| IBIS file stm32h523_533_ufbga100.ibs
[IBIS ver] 4.2
[File name] stm32h523_533_ufbga100.ibs
[File Rev] 0.2
[Date] 07-05-2024
[Source] Data Created at STMicroelectronics
[Notes]  File originated from ELDO simulations.
[Disclaimer]  This information is for modeling purpose only and is
   not guaranteed. The information is subject to change without
   notice.
[Copyright] Copyright 2024 STMicroelectronics Inc.
|   Component stm32h523_533_ufbga100
[Component] stm32h523_533_ufbga100
[Manufacturer] STMicroelectronics
[Package]
| variable   typ   min   max
R_pkg  0  NA  NA
L_pkg  0  NA  NA
C_pkg  0  NA  NA
[Pin]   signal_name   model_name
A1  PB9  io8_ft_i3c_spi
A2  PB8  io8_ft_i3c_spi
A3  BOOT0  vpphv
A4  PB5  io8_ft_i3c_spi
A5  PB3  io8_ft_i3c_spi
A6  PD6  io8_ft_i3c_spi
A7  PD4  io8_ft_i3c_spi
A8  PD3  io8_ft_i3c_spi
A9  PD1  io8_ft_i3c_spi
A10  PC11  io8_ft_i3c_spi
A11  PA15  io8_ft_i3c_spi
A12  PC10  io8_ft_i3c_spi
B1  PE0  io8_ft_i3c_spi
B2  PE4  io8_ft_i3c_spi
B3  PE3  io8_ft_i3c_spi
B4  PB6  io8_ft_i3c_spi
B5  PB4  io8_ft_i3c_spi
B6  PD7  io8_ft_i3c_spi
B7  PD5  io8_ft_i3c_spi
B8  PD2  io8_ft_i3c_spi
B9  PD0  io8_ft_i3c_spi
B10  PC12  io8_ft_i3c_spi
B11  PA14  io8_ft_i3c_spi
B12  PA13  io8_ft_i3c_spi
C1  PE2  io8_ft_i3c_spi
C2  PE5  io8_ft_i3c_spi
C3  VSS  gnd
C4  VCAP  nc
C5  PB7  io8_ft_i3c_spi
C8  VDDIO2  power
C9  VSS  gnd
C10  VDDUSB  power
C11  PA12  io8usb_ft_i3c_spi_phy
C12  PA11  io8usb_ft_i3c_spi_phy
D1  VBAT  power
D2  PE6  io8_ft_i3c_spi
D3  VDD  power
D10  VDD  power
D11  PA10  io8_ft_i3c_spi
D12  PA9  io8_ft_i3c_spi
E1  PC14-OSC32_IN  io_ft_tamp
E2  PC15-OSC32_OUT  io_ft_tamp
E3  PC13  io8_ft_i3c_spi_v33
E10  PA8  io8_ft_i3c_spi
E11  PC9  io8_ft_i3c_spi
E12  PC8  io8_ft_i3c_spi
F1  PH0-OSC_IN  io8_ft_i3c_spi
F2  PH1-OSC_OUT  io8_ft_i3c_spi
F11  PC7  io8_ft_i3c_spi
F12  PC6  io8_ft_i3c_spi
G1  PC0  io8_ft_spi
G2  NRST  ioreset_ft_v33
G11  PD14  io8_ft_i3c_spi
G12  PD15  io8_ft_i3c_spi
H1  PC2  io8_ft_spi
H2  PC3  io8_ft_spi
H3  PC1  io8_ft_spi
H10  PD11  io8_ft_i3c_spi
H11  PD12  io8_ft_i3c_spi
H12  PD13  io8_ft_i3c_spi
J1  VREFP  nc
J2  VSSA  nc
J3  VDD  power
J10  VDD  power
J11  PD9  io8_ft_i3c_spi
J12  PD10  io8_ft_i3c_spi
K1  VDDA  nc
K2  PA1  io8_ft_spi_tamp
K3  VSS  gnd
K4  PA2  io8_ft_spi
K5  PB1  io8_ft_spi
K8  PE12  io8_ft_i3c_spi
K9  VCAP  nc
K10  VSS  gnd
K11  PB14  nc
K12  PD8  io8_ft_i3c_spi
L1  PA3  io8_ft_spi
L2  PA4  io8_ft_spi
L3  PA0  io8_ft_spi
L4  PA7  io8_ft_spi
L5  PB2  io8_ft_i3c_spi
L6  VDD  power
L7  VSS  gnd
L8  PE10  io8_ft_i3c_spi
L9  PE13  io8_ft_i3c_spi
L10  PE15  io8_ft_i3c_spi
L11  PB12  io8_ft_i3c_spi
L12  PB15  io8_ft_spi
M1  PA6  io8_ft_spi
M2  PA5  io8_ft_spi
M3  PC4  io8_ft_spi
M4  PC5  io8_ft_spi
M5  PB0  io8_ft_spi
M6  PE7  io8_ft_i3c_spi
M7  PE8  io8_ft_i3c_spi
M8  PE9  io8_ft_i3c_spi
M9  PE11  io8_ft_i3c_spi
M10  PE14  io8_ft_i3c_spi
M11  PB10  io8_ft_i3c_spi
M12  PB13  nc
[Package Model]   478-ufbga7x7-100-240126
[Pin Mapping]   pulldown_ref   pullup_ref   | Comment
A1  gndio  vddmmc
A2  gndio  vddmmc
A3  gndio  vddio
A4  gndio  vddio
A5  gndio  vddio
A6  gndio  vddmmc
A7  gndio  vddio
A8  gndio  vddio
A9  gndio  vddio
A10  gndio  vddio
A11  gndio  vddio
A12  gndio  vddio
B1  gndio  vddio
B2  gndio  vddio
B3  gndio  vddio
B4  gndio  vddio
B5  gndio  vddio
B6  gndio  vddmmc
B7  gndio  vddio
B8  gndio  vddio
B9  gndio  vddio
B10  gndio  vddio
B11  gndio  vddio
B12  gndio  vddio
C1  gndio  vddio
C2  gndio  vddio
C3  gndio  nc
C4  nc  nc
C5  gndio  vddio
C8  nc  vddmmc
C9  gndio  nc
C10  nc  vddusb
C11  gndio  vddusb  | Depending on IO usage
| C11  gndio  vddio  | Depending on IO usage
C12  gndio  vddusb  | Depending on IO usage
| C12  gndio  vddio  | Depending on IO usage
D1  nc  vsw
D2  gndio  vddio
D3  nc  vddio
D10  nc  vddio
D11  gndio  vddio
D12  gndio  vddio
E1  gndio  vddio  | Depending on IO usage
| E1  gndio  vsw  | Depending on IO usage
E2  gndio  vddio  | Depending on IO usage
| E2  gndio  vsw  | Depending on IO usage
E3  gndio  vddio  | Depending on IO usage
| E3  gndio  vsw  | Depending on IO usage
E10  gndio  vddio
E11  gndio  vddio
E12  gndio  vddio
F1  gndio  vddio
F2  gndio  vddio
F11  gndio  vddio
F12  gndio  vddio
G1  gndio  vddio
G2  gndio  vddio
G11  gndio  vddio
G12  gndio  vddio
H1  gndio  vddio
H2  gndio  vddio
H3  gndio  vddio
H10  gndio  vddio
H11  gndio  vddio
H12  gndio  vddio
J1  nc  nc
J2  nc  nc
J3  nc  vddio
J10  nc  vddio
J11  gndio  vddio
J12  gndio  vddio
K1  nc  nc
K2  gndio  vddio
K3  gndio  nc
K4  gndio  vddio
K5  gndio  vddio
K8  gndio  vddio
K9  nc  nc
K10  gndio  nc
K11  nc  nc
K12  gndio  vddio
L1  gndio  vddio
L2  gndio  vddio
L3  gndio  vddio
L4  gndio  vddio
L5  gndio  vddio
L6  nc  vddio
L7  gndio  nc
L8  gndio  vddio
L9  gndio  vddio
L10  gndio  vddio
L11  gndio  vddio
L12  gndio  vddio
M1  gndio  vddio
M2  gndio  vddio
M3  gndio  vddio
M4  gndio  vddio
M5  gndio  vddio
M6  gndio  vddio
M7  gndio  vddio
M8  gndio  vddio
M9  gndio  vddio
M10  gndio  vddio
M11  gndio  vddio
M12  nc  nc
|[Diff Pin]  inv_pin  vdiff  tdelay_typ  tdelay_min  tdelay_max
|C11  C12  NA  NA  NA  NA
[Model Selector] io8_ft_i3c_spi
io8_ft_spi_ls_1v2 "GPIO SPI - 5V tolerant - low speed - 1.2V range"
io8_ft_spi_ls_1v8 "GPIO SPI - 5V tolerant - low speed - 1.8V range"
io8_ft_spi_ls_3v3 "GPIO SPI - 5V tolerant - low speed - 3.3V range"
io8_ft_spi_ms_1v2 "GPIO SPI - 5V tolerant - med speed - 1.2V range"
io8_ft_spi_ms_1v8 "GPIO SPI - 5V tolerant - med speed - 1.8V range"
io8_ft_spi_ms_3v3 "GPIO SPI - 5V tolerant - med speed - 3.3V range"
io8_ft_spi_fs_1v2 "GPIO SPI - 5V tolerant - fast speed - 1.2V range"
io8_ft_spi_fs_1v8 "GPIO SPI - 5V tolerant - fast speed - 1.8V range"
io8_ft_spi_fs_3v3 "GPIO SPI - 5V tolerant - fast speed - 3.3V range"
io8_ft_spi_hs_1v2 "GPIO SPI - 5V tolerant - high speed - 1.2V range"
io8_ft_spi_hs_1v8 "GPIO SPI - 5V tolerant - high speed - 1.8V range"
io8_ft_spi_hs_3v3 "GPIO SPI - 5V tolerant - high speed - 3.3V range"
io8_ft_hslv_spi_ls_1v2 "GPIO SPI low volt opt - 5V tolerant - low speed - 1.2V range"
io8_ft_hslv_spi_ls_1v8 "GPIO SPI low volt opt - 5V tolerant - low speed - 1.8V range"
io8_ft_hslv_spi_ls_2v5 "GPIO SPI low volt opt - 5V tolerant - low speed - 2.5V range"
io8_ft_hslv_spi_ms_1v2 "GPIO SPI low volt opt - 5V tolerant - med speed - 1.2V range"
io8_ft_hslv_spi_ms_1v8 "GPIO SPI low volt opt - 5V tolerant - med speed - 1.8V range"
io8_ft_hslv_spi_ms_2v5 "GPIO SPI low volt opt - 5V tolerant - med speed - 2.5V range"
io8_ft_hslv_spi_fs_1v2 "GPIO SPI low volt opt - 5V tolerant - fast speed - 1.2V range"
io8_ft_hslv_spi_fs_1v8 "GPIO SPI low volt opt - 5V tolerant - fast speed - 1.8V range"
io8_ft_hslv_spi_fs_2v5 "GPIO SPI low volt opt - 5V tolerant - fast speed - 2.5V range"
io8_ft_hslv_spi_hs_1v2 "GPIO SPI low volt opt - 5V tolerant - high speed - 1.2V range"
io8_ft_hslv_spi_hs_1v8 "GPIO SPI low volt opt - 5V tolerant - high speed - 1.8V range"
io8_ft_hslv_spi_hs_2v5 "GPIO SPI low volt opt - 5V tolerant - high speed - 2.5V range"
io8_ft_i3c_spi_ls_1v2 "GPIO SPI with I3C open-drain - 5V tolerant - low speed - 1.2V range"
io8_ft_i3c_spi_ls_1v8 "GPIO SPI with I3C open-drain - 5V tolerant - low speed - 1.8V range"
io8_ft_i3c_spi_ls_3v3 "GPIO SPI with I3C open-drain - 5V tolerant - low speed - 3.3V range"
io8_ft_i3c_spi_ms_1v2 "GPIO SPI with I3C open-drain - 5V tolerant - med speed - 1.2V range"
io8_ft_i3c_spi_ms_1v8 "GPIO SPI with I3C open-drain - 5V tolerant - med speed - 1.8V range"
io8_ft_i3c_spi_ms_3v3 "GPIO SPI with I3C open-drain - 5V tolerant - med speed - 3.3V range"
io8_ft_i3c_spi_fs_1v2 "GPIO SPI with I3C open-drain - 5V tolerant - fast speed - 1.2V range"
io8_ft_i3c_spi_fs_1v8 "GPIO SPI with I3C open-drain - 5V tolerant - fast speed - 1.8V range"
io8_ft_i3c_spi_fs_3v3 "GPIO SPI with I3C open-drain - 5V tolerant - fast speed - 3.3V range"
io8_ft_i3c_spi_hs_1v2 "GPIO SPI with I3C open-drain - 5V tolerant - high speed - 1.2V range"
io8_ft_i3c_spi_hs_1v8 "GPIO SPI with I3C open-drain - 5V tolerant - high speed - 1.8V range"
io8_ft_i3c_spi_hs_3v3 "GPIO SPI with I3C open-drain - 5V tolerant - high speed - 3.3V range"
io8_ft_hslv_i3c_spi_ls_1v2 "GPIO SPI low volt opt with I3C open-drain - 5V tolerant - low speed - 1.2V range"
io8_ft_hslv_i3c_spi_ls_1v8 "GPIO SPI low volt opt with I3C open-drain - 5V tolerant - low speed - 1.8V range"
io8_ft_hslv_i3c_spi_ls_2v5 "GPIO SPI low volt opt with I3C open-drain - 5V tolerant - low speed - 2.5V range"
io8_ft_hslv_i3c_spi_ms_1v2 "GPIO SPI low volt opt with I3C open-drain - 5V tolerant - med speed - 1.2V range"
io8_ft_hslv_i3c_spi_ms_1v8 "GPIO SPI low volt opt with I3C open-drain - 5V tolerant - med speed - 1.8V range"
io8_ft_hslv_i3c_spi_ms_2v5 "GPIO SPI low volt opt with I3C open-drain - 5V tolerant - med speed - 2.5V range"
io8_ft_hslv_i3c_spi_fs_1v2 "GPIO SPI low volt opt with I3C open-drain - 5V tolerant - fast speed - 1.2V range"
io8_ft_hslv_i3c_spi_fs_1v8 "GPIO SPI low volt opt with I3C open-drain - 5V tolerant - fast speed - 1.8V range"
io8_ft_hslv_i3c_spi_fs_2v5 "GPIO SPI low volt opt with I3C open-drain - 5V tolerant - fast speed - 2.5V range"
io8_ft_hslv_i3c_spi_hs_1v2 "GPIO SPI low volt opt with I3C open-drain - 5V tolerant - high speed - 1.2V range"
io8_ft_hslv_i3c_spi_hs_1v8 "GPIO SPI low volt opt with I3C open-drain - 5V tolerant - high speed - 1.8V range"
io8_ft_hslv_i3c_spi_hs_2v5 "GPIO SPI low volt opt with I3C open-drain - 5V tolerant - high speed - 2.5V range"
io8_ft_i3c_fmp_spi_3v3 "GPIO SPI with I3C fm+ open-drain - 5V tolerant - 3.3V range"
io8_ft_i3c_fmp_spi_1v8 "GPIO SPI with I3C fm+ open-drain - 5V tolerant - 1.8V range"
io8_ft_i3c_fmp_spi_1v2 "GPIO SPI with I3C fm+ open-drain - 5V tolerant - 1.2V range"
[Model Selector] io8_ft_i3c_spi_v33
io8_ft_spi_v33_ls_1v2 ""GPIO SPI V33 - 5V tolerant - low speed - 1.2V range"
io8_ft_spi_v33_ls_1v8 ""GPIO SPI V33 - 5V tolerant - low speed - 1.8V range"
io8_ft_spi_v33_ls_3v3 ""GPIO SPI V33 - 5V tolerant - low speed - 3.3V range"
io8_ft_spi_v33_ms_1v2 ""GPIO SPI V33 - 5V tolerant - med speed - 1.2V range"
io8_ft_spi_v33_ms_1v8 ""GPIO SPI V33 - 5V tolerant - med speed - 1.8V range"
io8_ft_spi_v33_ms_3v3 ""GPIO SPI V33 - 5V tolerant - med speed - 3.3V range"
io8_ft_spi_v33_fs_1v2 ""GPIO SPI V33 - 5V tolerant - fast speed - 1.2V range
io8_ft_spi_v33_fs_1v8 ""GPIO SPI V33 - 5V tolerant - fast speed - 1.8V range
io8_ft_spi_v33_fs_3v3 ""GPIO SPI V33 - 5V tolerant - fast speed - 3.3V range
io8_ft_spi_v33_hs_1v2 ""GPIO SPI V33 - 5V tolerant - high speed - 1.2V range
io8_ft_spi_v33_hs_1v8 ""GPIO SPI V33 - 5V tolerant - high speed - 1.8V range
io8_ft_spi_v33_hs_3v3 ""GPIO SPI V33 - 5V tolerant - high speed - 3.3V range
io8_ft_hslv_spi_v33_ls_1v2 "GPIO SPI V33 low volt opt - 5V tolerant - low speed - 1.2V range""
io8_ft_hslv_spi_v33_ls_1v8 "GPIO SPI V33 low volt opt - 5V tolerant - low speed - 1.8V range""
io8_ft_hslv_spi_v33_ls_2v5 "GPIO SPI V33 low volt opt - 5V tolerant - low speed - 2.5V range""
io8_ft_hslv_spi_v33_ms_1v2 "GPIO SPI V33 low volt opt - 5V tolerant - med speed - 1.2V range""
io8_ft_hslv_spi_v33_ms_1v8 "GPIO SPI V33 low volt opt - 5V tolerant - med speed - 1.8V range""
io8_ft_hslv_spi_v33_ms_2v5 "GPIO SPI V33 low volt opt - 5V tolerant - med speed - 2.5V range""
io8_ft_hslv_spi_v33_fs_1v2 "GPIO SPI V33 low volt opt - 5V tolerant - fast speed - 1.2V range"
io8_ft_hslv_spi_v33_fs_1v8 "GPIO SPI V33 low volt opt - 5V tolerant - fast speed - 1.8V range"
io8_ft_hslv_spi_v33_fs_2v5 "GPIO SPI V33 low volt opt - 5V tolerant - fast speed - 2.5V range"
io8_ft_hslv_spi_v33_hs_1v2 "GPIO SPI V33 low volt opt - 5V tolerant - high speed - 1.2V range"
io8_ft_hslv_spi_v33_hs_1v8 "GPIO SPI V33 low volt opt - 5V tolerant - high speed - 1.8V range"
io8_ft_hslv_spi_v33_hs_2v5 "GPIO SPI V33 low volt opt - 5V tolerant - high speed - 2.5V range"
io8_ft_i3c_spi_v33_ls_1v2 "GPIO SPI V33 with I3C open-drain - 5V tolerant - low speed - 1.2V range"
io8_ft_i3c_spi_v33_ls_1v8 "GPIO SPI V33 with I3C open-drain - 5V tolerant - low speed - 1.8V range"
io8_ft_i3c_spi_v33_ls_3v3 "GPIO SPI V33 with I3C open-drain - 5V tolerant - low speed - 3.3V range"
io8_ft_i3c_spi_v33_ms_1v2 "GPIO SPI V33 with I3C open-drain - 5V tolerant - med speed - 1.2V range"
io8_ft_i3c_spi_v33_ms_1v8 "GPIO SPI V33 with I3C open-drain - 5V tolerant - med speed - 1.8V range"
io8_ft_i3c_spi_v33_ms_3v3 "GPIO SPI V33 with I3C open-drain - 5V tolerant - med speed - 3.3V range"
io8_ft_i3c_spi_v33_fs_1v2 "GPIO SPI V33 with I3C open-drain - 5V tolerant - fast speed - 1.2V range"
io8_ft_i3c_spi_v33_fs_1v8 "GPIO SPI V33 with I3C open-drain - 5V tolerant - fast speed - 1.8V range"
io8_ft_i3c_spi_v33_fs_3v3 "GPIO SPI V33 with I3C open-drain - 5V tolerant - fast speed - 3.3V range"
io8_ft_i3c_spi_v33_hs_1v2 "GPIO SPI V33 with I3C open-drain - 5V tolerant - high speed - 1.2V range"
io8_ft_i3c_spi_v33_hs_1v8 "GPIO SPI V33 with I3C open-drain - 5V tolerant - high speed - 1.8V range"
io8_ft_i3c_spi_v33_hs_3v3 "GPIO SPI V33 with I3C open-drain - 5V tolerant - high speed - 3.3V range"
io8_ft_hslv_i3c_spi_v33_ls_1v2 "GPIO SPI V33 low volt opt with I3C open-drain - 5V tolerant - low speed - 1.2V range"
io8_ft_hslv_i3c_spi_v33_ls_1v8 "GPIO SPI V33 low volt opt with I3C open-drain - 5V tolerant - low speed - 1.8V range"
io8_ft_hslv_i3c_spi_v33_ls_2v5 "GPIO SPI V33 low volt opt with I3C open-drain - 5V tolerant - low speed - 2.5V range"
io8_ft_hslv_i3c_spi_v33_ms_1v2 "GPIO SPI V33 low volt opt with I3C open-drain - 5V tolerant - med speed - 1.2V range"
io8_ft_hslv_i3c_spi_v33_ms_1v8 "GPIO SPI V33 low volt opt with I3C open-drain - 5V tolerant - med speed - 1.8V range"
io8_ft_hslv_i3c_spi_v33_ms_2v5 "GPIO SPI V33 low volt opt with I3C open-drain - 5V tolerant - med speed - 2.5V range"
io8_ft_hslv_i3c_spi_v33_fs_1v2 "GPIO SPI V33 low volt opt with I3C open-drain - 5V tolerant - fast speed - 1.2V range"
io8_ft_hslv_i3c_spi_v33_fs_1v8 "GPIO SPI V33 low volt opt with I3C open-drain - 5V tolerant - fast speed - 1.8V range"
io8_ft_hslv_i3c_spi_v33_fs_2v5 "GPIO SPI V33 low volt opt with I3C open-drain - 5V tolerant - fast speed - 2.5V range"
io8_ft_hslv_i3c_spi_v33_hs_1v2 "GPIO SPI V33 low volt opt with I3C open-drain - 5V tolerant - high speed - 1.2V range"
io8_ft_hslv_i3c_spi_v33_hs_1v8 "GPIO SPI V33 low volt opt with I3C open-drain - 5V tolerant - high speed - 1.8V range"
io8_ft_hslv_i3c_spi_v33_hs_2v5 "GPIO SPI V33 low volt opt with I3C open-drain - 5V tolerant - high speed - 2.5V range"
io8_ft_i3c_fmp_spi_v33_3v3 "GPIO SPI V33 with I3C fm+ open-drain - 5V tolerant - 3.3V range"
io8_ft_i3c_fmp_spi_v33_1v8 "GPIO SPI V33 with I3C fm+ open-drain - 5V tolerant - 1.8V range"
io8_ft_i3c_fmp_spi_v33_1v2 "GPIO SPI V33 with I3C fm+ open-drain - 5V tolerant - 1.2V range"
[Model Selector] io8_ft_spi
io8_ft_spi_ls_1v2 "GPIO SPI - 5V tolerant - low speed - 1.2V range"
io8_ft_spi_ls_1v8 "GPIO SPI - 5V tolerant - low speed - 1.8V range"
io8_ft_spi_ls_3v3 "GPIO SPI - 5V tolerant - low speed - 3.3V range"
io8_ft_spi_ms_1v2 "GPIO SPI- 5V tolerant - med speed - 1.2V range"
io8_ft_spi_ms_1v8 "GPIO SPI- 5V tolerant - med speed - 1.8V range"
io8_ft_spi_ms_3v3 "GPIO SPI- 5V tolerant - med speed - 3.3V range"
io8_ft_spi_fs_1v2 "GPIO SPI- 5V tolerant - fast speed - 1.2V range"
io8_ft_spi_fs_1v8 "GPIO SPI- 5V tolerant - fast speed - 1.8V range"
io8_ft_spi_fs_3v3 "GPIO SPI- 5V tolerant - fast speed - 3.3V range"
io8_ft_spi_hs_1v2 "GPIO SPI- 5V tolerant - high speed - 1.2V range"
io8_ft_spi_hs_1v8 "GPIO SPI- 5V tolerant - high speed - 1.8V range"
io8_ft_spi_hs_3v3 "GPIO SPI- 5V tolerant - high speed - 3.3V range"
io8_ft_hslv_spi_ls_1v2 "GPIO SPI low volt opt - 5V tolerant - low speed - 1.2V range"
io8_ft_hslv_spi_ls_1v8 "GPIO SPI low volt opt - 5V tolerant - low speed - 1.8V range"
io8_ft_hslv_spi_ls_2v5 "GPIO SPI low volt opt - 5V tolerant - low speed - 2.5V range"
io8_ft_hslv_spi_ms_1v2 "GPIO SPI low volt opt - 5V tolerant - med speed - 1.2V range"
io8_ft_hslv_spi_ms_1v8 "GPIO SPI low volt opt - 5V tolerant - med speed - 1.8V range"
io8_ft_hslv_spi_ms_2v5 "GPIO SPI low volt opt - 5V tolerant - med speed - 2.5V range"
io8_ft_hslv_spi_fs_1v2 "GPIO SPI low volt opt - 5V tolerant - fast speed - 1.2V range"
io8_ft_hslv_spi_fs_1v8 "GPIO SPI low volt opt - 5V tolerant - fast speed - 1.8V range"
io8_ft_hslv_spi_fs_2v5 "GPIO SPI low volt opt - 5V tolerant - fast speed - 2.5V range"
io8_ft_hslv_spi_hs_1v2 "GPIO SPI low volt opt - 5V tolerant - high speed - 1.2V range"
io8_ft_hslv_spi_hs_1v8 "GPIO SPI low volt opt - 5V tolerant - high speed - 1.8V range"
io8_ft_hslv_spi_hs_2v5 "GPIO SPI low volt opt - 5V tolerant - high speed - 2.5V range"
[Model Selector] io8_ft_spi_tamp
io8_ft_spi_ls_1v2 "GPIO SPI - 5V tolerant - low speed - 1.2V range"
io8_ft_spi_ls_1v8 "GPIO SPI - 5V tolerant - low speed - 1.8V range"
io8_ft_spi_ls_3v3 "GPIO SPI- 5V tolerant - low speed - 3.3V range"
io8_ft_spi_ms_1v2 "GPIO SPI - 5V tolerant - med speed - 1.2V range"
io8_ft_spi_ms_1v8 "GPIO SPI - 5V tolerant - med speed - 1.8V range"
io8_ft_spi_ms_3v3 "GPIO SPI - 5V tolerant - med speed - 3.3V range"
io8_ft_spi_fs_1v2 "GPIO SPI - 5V tolerant - fast speed - 1.2V range"
io8_ft_spi_fs_1v8 "GPIO SPI - 5V tolerant - fast speed - 1.8V range"
io8_ft_spi_fs_3v3 "GPIO SPI - 5V tolerant - fast speed - 3.3V range"
io8_ft_spi_hs_1v2 "GPIO SPI - 5V tolerant - high speed - 1.2V range"
io8_ft_spi_hs_1v8 "GPIO SPI - 5V tolerant - high speed - 1.8V range"
io8_ft_spi_hs_3v3 "GPIO SPI - 5V tolerant - high speed - 3.3V range"
io8_ft_hslv_spi_ls_1v2 "GPIO SPI low volt opt - 5V tolerant - low speed - 1.2V range"
io8_ft_hslv_spi_ls_1v8 "GPIO SPI low volt opt - 5V tolerant - low speed - 1.8V range"
io8_ft_hslv_spi_ls_2v5 "GPIO SPI low volt opt - 5V tolerant - low speed - 2.5V range"
io8_ft_hslv_spi_ms_1v2 "GPIO SPI low volt opt - 5V tolerant - med speed - 1.2V range"
io8_ft_hslv_spi_ms_1v8 "GPIO SPI low volt opt - 5V tolerant - med speed - 1.8V range"
io8_ft_hslv_spi_ms_2v5 "GPIO SPI low volt opt - 5V tolerant - med speed - 2.5V range"
io8_ft_hslv_spi_fs_1v2 "GPIO SPI low volt opt - 5V tolerant - fast speed - 1.2V range"
io8_ft_hslv_spi_fs_1v8 "GPIO SPI low volt opt - 5V tolerant - fast speed - 1.8V range"
io8_ft_hslv_spi_fs_2v5 "GPIO SPI low volt opt - 5V tolerant - fast speed - 2.5V range"
io8_ft_hslv_spi_hs_1v2 "GPIO SPI low volt opt - 5V tolerant - high speed - 1.2V range"
io8_ft_hslv_spi_hs_1v8 "GPIO SPI low volt opt - 5V tolerant - high speed - 1.8V range"
io8_ft_hslv_spi_hs_2v5 "GPIO SPI low volt opt - 5V tolerant - high speed - 2.5V range
io8_ft_tamp_v33_1v2 "IO tamper - 5V tolerant - 1.2V range"
io8_ft_tamp_v33_1v8 "IO tamper - 5V tolerant - 1.8V range"
io8_ft_tamp_v33_3v3 "IO tamper - 5V tolerant - 3.3V range"
[Model Selector] io8usb_ft_i3c_spi_phy
io8_ft_spi_ls_1v2 "GPIO SPI - 5V tolerant - low speed - 1.2V range"
io8_ft_spi_ls_1v8 "GPIO SPI - 5V tolerant - low speed - 1.8V range"
io8_ft_spi_ls_3v3 "GPIO SPI - 5V tolerant - low speed - 3.3V range"
io8_ft_spi_ms_1v2 "GPIO SPI - 5V tolerant - med speed - 1.2V range"
io8_ft_spi_ms_1v8 "GPIO SPI - 5V tolerant - med speed - 1.8V range"
io8_ft_spi_ms_3v3 "GPIO SPI - 5V tolerant - med speed - 3.3V range"
io8_ft_spi_fs_1v2 "GPIO SPI - 5V tolerant - fast speed - 1.2V range"
io8_ft_spi_fs_1v8 "GPIO SPI - 5V tolerant - fast speed - 1.8V range"
io8_ft_spi_fs_3v3 "GPIO SPI - 5V tolerant - fast speed - 3.3V range"
io8_ft_spi_hs_1v2 "GPIO SPI - 5V tolerant - high speed - 1.2V range"
io8_ft_spi_hs_1v8 "GPIO SPI - 5V tolerant - high speed - 1.8V range"
io8_ft_spi_hs_3v3 "GPIO SPI - 5V tolerant - high speed - 3.3V range"
io8_ft_hslv_spi_ls_1v2 "GPIO SPI low volt opt - 5V tolerant - low speed - 1.2V range"
io8_ft_hslv_spi_ls_1v8 "GPIO SPI low volt opt - 5V tolerant - low speed - 1.8V range"
io8_ft_hslv_spi_ls_2v5 "GPIO SPI low volt opt - 5V tolerant - low speed - 2.5V range"
io8_ft_hslv_spi_ms_1v2 "GPIO SPI low volt opt - 5V tolerant - med speed - 1.2V range"
io8_ft_hslv_spi_ms_1v8 "GPIO SPI low volt opt - 5V tolerant - med speed - 1.8V range"
io8_ft_hslv_spi_ms_2v5 "GPIO SPI low volt opt - 5V tolerant - med speed - 2.5V range"
io8_ft_hslv_spi_fs_1v2 "GPIO SPI low volt opt - 5V tolerant - fast speed - 1.2V range"
io8_ft_hslv_spi_fs_1v8 "GPIO SPI low volt opt - 5V tolerant - fast speed - 1.8V range"
io8_ft_hslv_spi_fs_2v5 "GPIO SPI low volt opt - 5V tolerant - fast speed - 2.5V range"
io8_ft_hslv_spi_hs_1v2 "GPIO SPI low volt opt - 5V tolerant - high speed - 1.2V range"
io8_ft_hslv_spi_hs_1v8 "GPIO SPI low volt opt - 5V tolerant - high speed - 1.8V range"
io8_ft_hslv_spi_hs_2v5 "GPIO SPI low volt opt - 5V tolerant - high speed - 2.5V range"
io8_ft_i3c_spi_ls_1v2 "GPIO SPI  with I3C open-drain - 5V tolerant - low speed - 1.2V range"
io8_ft_i3c_spi_ls_1v8 "GPIO SPI  with I3C open-drain - 5V tolerant - low speed - 1.8V range"
io8_ft_i3c_spi_ls_3v3 "GPIO SPI  with I3C open-drain - 5V tolerant - low speed - 3.3V range"
io8_ft_i3c_spi_ms_1v2 "GPIO SPI  with I3C open-drain - 5V tolerant - med speed - 1.2V range"
io8_ft_i3c_spi_ms_1v8 "GPIO SPI  with I3C open-drain - 5V tolerant - med speed - 1.8V range"
io8_ft_i3c_spi_ms_3v3 "GPIO SPI  with I3C open-drain - 5V tolerant - med speed - 3.3V range"
io8_ft_i3c_spi_fs_1v2 "GPIO SPI  with I3C open-drain - 5V tolerant - fast speed - 1.2V range"
io8_ft_i3c_spi_fs_1v8 "GPIO SPI  with I3C open-drain - 5V tolerant - fast speed - 1.8V range"
io8_ft_i3c_spi_fs_3v3 "GPIO SPI  with I3C open-drain - 5V tolerant - fast speed - 3.3V range"
io8_ft_i3c_spi_hs_1v2 "GPIO SPI  with I3C open-drain - 5V tolerant - high speed - 1.2V range"
io8_ft_i3c_spi_hs_1v8 "GPIO SPI  with I3C open-drain - 5V tolerant - high speed - 1.8V range"
io8_ft_i3c_spi_hs_3v3 "GPIO SPI  with I3C open-drain - 5V tolerant - high speed - 3.3V range"
io8_ft_hslv_i3c_spi_ls_1v2 "GPIO SPI  low volt opt with I3C open-drain - 5V tolerant - low speed - 1.2V range"
io8_ft_hslv_i3c_spi_ls_1v8 "GPIO SPI  low volt opt with I3C open-drain - 5V tolerant - low speed - 1.8V range"
io8_ft_hslv_i3c_spi_ls_2v5 "GPIO SPI  low volt opt with I3C open-drain - 5V tolerant - low speed - 2.5V range"
io8_ft_hslv_i3c_spi_ms_1v2 "GPIO SPI  low volt opt with I3C open-drain - 5V tolerant - med speed - 1.2V range"
io8_ft_hslv_i3c_spi_ms_1v8 "GPIO SPI  low volt opt with I3C open-drain - 5V tolerant - med speed - 1.8V range"
io8_ft_hslv_i3c_spi_ms_2v5 "GPIO SPI  low volt opt with I3C open-drain - 5V tolerant - med speed - 2.5V range"
io8_ft_hslv_i3c_spi_fs_1v2 "GPIO SPI  low volt opt with I3C open-drain - 5V tolerant - fast speed - 1.2V range"
io8_ft_hslv_i3c_spi_fs_1v8 "GPIO SPI  low volt opt with I3C open-drain - 5V tolerant - fast speed - 1.8V range"
io8_ft_hslv_i3c_spi_fs_2v5 "GPIO SPI  low volt opt with I3C open-drain - 5V tolerant - fast speed - 2.5V range"
io8_ft_hslv_i3c_spi_hs_1v2 "GPIO SPI  low volt opt with I3C open-drain - 5V tolerant - high speed - 1.2V range"
io8_ft_hslv_i3c_spi_hs_1v8 "GPIO SPI  low volt opt with I3C open-drain - 5V tolerant - high speed - 1.8V range"
io8_ft_hslv_i3c_spi_hs_2v5 "GPIO SPI  low volt opt with I3C open-drain - 5V tolerant - high speed - 2.5V range"
io8_ft_i3c_fmp_spi_3v3 "GPIO SPI  with I3C fm+ open-drain - 5V tolerant - 3.3V range"
io8_ft_i3c_fmp_spi_1v8 "GPIO SPI  with I3C fm+ open-drain - 5V tolerant - 1.8V range"
io8_ft_i3c_fmp_spi_1v2 "GPIO SPI  with I3C fm+ open-drain - 5V tolerant - 1.2V range"
io8usb_ft_phy_ls_2v5 "USB PHY - 5V tolerant - low speed - 2.5V range"
io8usb_ft_phy_ls_3v3 "USB PHY - 5V tolerant - low speed - 3.3V range
io8usb_ft_phy_fs_2v5 "USB PHY - 5V tolerant - fast speed - 2.5V range"
io8usb_ft_phy_fs_3v3 "USB PHY - 5V tolerant - fast speed - 3.3V range"
[Model Selector] io_ft_tamp
io_ft_tamp_3v3 "IO tamper - 5V tolerant - 3.3V range"
io_ft_tamp_1v8 "IO tamper - 5V tolerant - 1.8V range"
io_ft_tamp_1v2 "IO tamper - 5V tolerant - 1.2V range"
[Model Selector] ioreset_ft_v33
ioreset_ft_v33_1v2 "Reset PAD. 5V tolerant. 1.2V range"
ioreset_ft_v33_1v8 "Reset PAD. 5V tolerant. 1.8V range"
ioreset_ft_v33_3v3 "Reset PAD. 5V tolerant. 3.3V range"
[Model Selector] vpphv
vpphv_1v2 "Flash Test cell v33 = 1.2 V range"
vpphv_1v8 "Flash Test cell v33 = 1.8 V range"
vpphv_3v3 "Flash Test cell v33 = 3.3 V range"
[Define Package Model]  478-ufbga7x7-100-240126
[Manufacturer]  unknown
[OEM]  unknown
[Description]  unknown
[Number Of Pins]  92
[Pin Numbers]
| Pin Name Terminal   Net Name   Starting Node   Ending Node
A3 | BOOT0
G2 | NRST
L3 | PA0
K2 | PA1
K4 | PA2
L1 | PA3
L2 | PA4
M2 | PA5
M1 | PA6
L4 | PA7
E10 | PA8
D12 | PA9
D11 | PA10
C12 | PA11
C11 | PA12
B12 | PA13
B11 | PA14
A11 | PA15
M5 | PB0
K5 | PB1
L5 | PB2
A5 | PB3
B5 | PB4
A4 | PB5
B4 | PB6
C5 | PB7
A2 | PB8
A1 | PB9
M11 | PB10
L11 | PB12
M12 | PB13
K11 | PB14
L12 | PB15
G1 | PC0
H3 | PC1
H1 | PC2
H2 | PC3
M3 | PC4
M4 | PC5
F12 | PC6
F11 | PC7
E12 | PC8
E11 | PC9
A12 | PC10
A10 | PC11
B10 | PC12
E3 | PC13
E1 | PC14-OSC32_IN
E2 | PC15-OSC32_OUT
B9 | PD0
A9 | PD1
B8 | PD2
A8 | PD3
A7 | PD4
B7 | PD5
A6 | PD6
B6 | PD7
K12 | PD8
J11 | PD9
J12 | PD10
H10 | PD11
H11 | PD12
H12 | PD13
G11 | PD14
G12 | PD15
B1 | PE0
C1 | PE2
B3 | PE3
B2 | PE4
C2 | PE5
D2 | PE6
M6 | PE7
M7 | PE8
M8 | PE9
L8 | PE10
M9 | PE11
K8 | PE12
L9 | PE13
M10 | PE14
L10 | PE15
F1 | PH0-OSC_IN
F2 | PH1-OSC_OUT
D1 | VBAT
K9 | VCAP
C4 | VCAP
D3 | VDD
K1 | VDDA
C8 | VDDIO2
C10 | VDDUSB
J1 | VREFP
C3 | VSS
J2 | VSSA
|[Merged Pins]  D3
|D10  |  VDD
|J3  |  VDD
|J10  |  VDD
|L6  |  VDD
|[Merged Pins]  C3
|C9  |  VSS
|K3  |  VSS
|K10  |  VSS
|L7  |  VSS
[Model Data]
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[End Model Data]
[End Package Model]
|End [Component]
| Models and submodels in the file (118): io8_ft_hslv_i3c_spi_fs_1v2 (I/O_open_drain), io8_ft_hslv_i3c_spi_fs_1v8 (I/O_open_drain), io8_ft_hslv_i3c_spi_fs_2v5 (I/O_open_drain), io8_ft_hslv_i3c_spi_hs_1v2 (I/O_open_drain), io8_ft_hslv_i3c_spi_hs_1v8 (I/O_open_drain), io8_ft_hslv_i3c_spi_hs_2v5 (I/O_open_drain), io8_ft_hslv_i3c_spi_ls_1v2 (I/O_open_drain), io8_ft_hslv_i3c_spi_ls_1v8 (I/O_open_drain), io8_ft_hslv_i3c_spi_ls_2v5 (I/O_open_drain), io8_ft_hslv_i3c_spi_ms_1v2 (I/O_open_drain), io8_ft_hslv_i3c_spi_ms_1v8 (I/O_open_drain), io8_ft_hslv_i3c_spi_ms_2v5 (I/O_open_drain), io8_ft_hslv_i3c_spi_v33_fs_1v2 (I/O_open_drain), io8_ft_hslv_i3c_spi_v33_fs_1v8 (I/O_open_drain), io8_ft_hslv_i3c_spi_v33_fs_2v5 (I/O_open_drain), io8_ft_hslv_i3c_spi_v33_hs_1v2 (I/O_open_drain), io8_ft_hslv_i3c_spi_v33_hs_1v8 (I/O_open_drain), io8_ft_hslv_i3c_spi_v33_hs_2v5 (I/O_open_drain), io8_ft_hslv_i3c_spi_v33_ls_1v2 (I/O_open_drain), io8_ft_hslv_i3c_spi_v33_ls_1v8 (I/O_open_drain), io8_ft_hslv_i3c_spi_v33_ls_2v5 (I/O_open_drain), io8_ft_hslv_i3c_spi_v33_ms_1v2 (I/O_open_drain), io8_ft_hslv_i3c_spi_v33_ms_1v8 (I/O_open_drain), io8_ft_hslv_i3c_spi_v33_ms_2v5 (I/O_open_drain), io8_ft_hslv_spi_fs_1v2 (I/O), io8_ft_hslv_spi_fs_1v8 (I/O), io8_ft_hslv_spi_fs_2v5 (I/O), io8_ft_hslv_spi_hs_1v2 (I/O), io8_ft_hslv_spi_hs_1v8 (I/O), io8_ft_hslv_spi_hs_2v5 (I/O), io8_ft_hslv_spi_ls_1v2 (I/O), io8_ft_hslv_spi_ls_1v8 (I/O), io8_ft_hslv_spi_ls_2v5 (I/O), io8_ft_hslv_spi_ms_1v2 (I/O), io8_ft_hslv_spi_ms_1v8 (I/O), io8_ft_hslv_spi_ms_2v5 (I/O), io8_ft_hslv_spi_v33_fs_1v2 (I/O), io8_ft_hslv_spi_v33_fs_1v8 (I/O), io8_ft_hslv_spi_v33_fs_2v5 (I/O), io8_ft_hslv_spi_v33_hs_1v2 (I/O), io8_ft_hslv_spi_v33_hs_1v8 (I/O), io8_ft_hslv_spi_v33_hs_2v5 (I/O), io8_ft_hslv_spi_v33_ls_1v2 (I/O), io8_ft_hslv_spi_v33_ls_1v8 (I/O), io8_ft_hslv_spi_v33_ls_2v5 (I/O), io8_ft_hslv_spi_v33_ms_1v2 (I/O), io8_ft_hslv_spi_v33_ms_1v8 (I/O), io8_ft_hslv_spi_v33_ms_2v5 (I/O), io8_ft_i3c_fmp_spi_1v2 (I/O_open_drain), io8_ft_i3c_fmp_spi_1v8 (I/O_open_drain), io8_ft_i3c_fmp_spi_3v3 (I/O_open_drain), io8_ft_i3c_fmp_spi_v33_1v2 (I/O_open_drain), io8_ft_i3c_fmp_spi_v33_1v8 (I/O_open_drain), io8_ft_i3c_fmp_spi_v33_3v3 (I/O_open_drain), io8_ft_i3c_spi_fs_1v2 (I/O_open_drain), io8_ft_i3c_spi_fs_1v8 (I/O_open_drain), io8_ft_i3c_spi_fs_3v3 (I/O_open_drain), io8_ft_i3c_spi_hs_1v2 (I/O_open_drain), io8_ft_i3c_spi_hs_1v8 (I/O_open_drain), io8_ft_i3c_spi_hs_3v3 (I/O_open_drain), io8_ft_i3c_spi_ls_1v2 (I/O_open_drain), io8_ft_i3c_spi_ls_1v8 (I/O_open_drain), io8_ft_i3c_spi_ls_3v3 (I/O_open_drain), io8_ft_i3c_spi_ms_1v2 (I/O_open_drain), io8_ft_i3c_spi_ms_1v8 (I/O_open_drain), io8_ft_i3c_spi_ms_3v3 (I/O_open_drain), io8_ft_i3c_spi_v33_fs_1v2 (I/O_open_drain), io8_ft_i3c_spi_v33_fs_1v8 (I/O_open_drain), io8_ft_i3c_spi_v33_fs_3v3 (I/O_open_drain), io8_ft_i3c_spi_v33_hs_1v2 (I/O_open_drain), io8_ft_i3c_spi_v33_hs_1v8 (I/O_open_drain), io8_ft_i3c_spi_v33_hs_3v3 (I/O_open_drain), io8_ft_i3c_spi_v33_ls_1v2 (I/O_open_drain), io8_ft_i3c_spi_v33_ls_1v8 (I/O_open_drain), io8_ft_i3c_spi_v33_ls_3v3 (I/O_open_drain), io8_ft_i3c_spi_v33_ms_1v2 (I/O_open_drain), io8_ft_i3c_spi_v33_ms_1v8 (I/O_open_drain), io8_ft_i3c_spi_v33_ms_3v3 (I/O_open_drain), io8_ft_spi_fs_1v2 (I/O), io8_ft_spi_fs_1v8 (I/O)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
